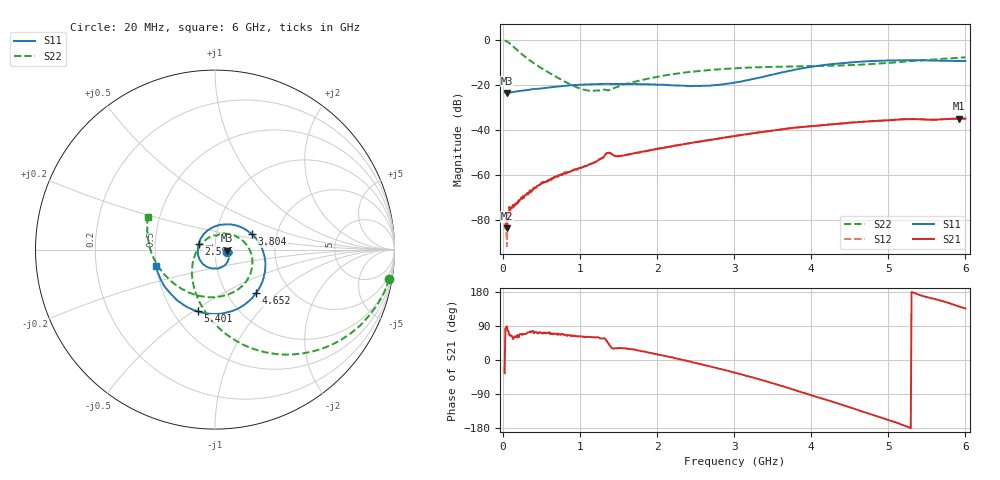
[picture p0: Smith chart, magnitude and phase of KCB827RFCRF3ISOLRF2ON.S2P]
!Agilent Technologies,E5071B,JP1KK00126,A.08.11
!Date: Tue May 06 07:21:44 2014
!Data & Calibration Information:
!Freq	S11:SOLT2(ON)	S21:SOLT2(ON)	S12:SOLT2(ON)	S22:SOLT2(ON)
# Hz S dB R 50
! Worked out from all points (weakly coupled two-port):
!   600 points, 20 MHz to 6 GHz, reference 50 ohm
!   highest |S21| = -34.86 dB at 5.92 GHz (marker M1); lowest = -83.7 dB at 49.95 MHz (marker M2)
!   lowest |S11| = -23.4 dB at 49.95 MHz (marker M3), VSWR 1.14, Z = 57.2 - j0.642 ohm
!   |S11| at or under -10 dB: start of sweep to 4.461 GHz
!   |S22| runs from -22.6 to -0.1 dB; largest |S21 - S12| = 0.00014
!   S11 on the Smith chart (normalised r, x): 20 MHz: 1.14, -0.03; 2.596 GHz: 0.83, +0.05; 3.804 GHz: 1.49, +0.27; 4.652 GHz: 1.36, -0.74; 5.401 GHz: 0.66, -0.52; 6 GHz: 0.50, -0.10
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2e7  -23.20 -12.7  -82.57 -34.7  -84.04 -22.6  -0.13 -9.6
4.994992e7  -23.43 -4.8  -83.69 88.9  -91.59 17.7  -0.60 -23.3
8.988314e7  -23.29 -3.3  -74.31 64.0  -78.09 80.3  -1.54 -39.4
1.397997e8  -23.01 -3.6  -73.86 59.9  -74.07 63.1  -3.04 -56.1
2.196661e8  -22.55 -5.7  -70.89 68.2  -71.16 69.3  -5.50 -75.9
3.294825e8  -22.12 -12.0  -68.46 73.3  -67.84 77.3  -8.55 -95.6
5.690818e8  -21.21 -25.9  -62.47 71.8  -62.66 69.4  -13.93 -129.2
1.018331e9  -19.75 -58.4  -56.70 62.5  -56.49 63.0  -21.78 157.1
1.19803e9  -19.55 -72.7  -54.10 59.7  -54.22 60.3  -22.44 116.5
1.357763e9  -19.45 -85.7  -50.19 45.8  -50.16 45.6  -22.24 84.8
1.517496e9  -19.46 -99.3  -51.44 31.6  -51.50 32.1  -20.35 66.8
2.016661e9  -19.82 -141.6  -48.24 14.4  -48.21 14.7  -16.20 21.7
2.595693e9  -20.27 161.2  -44.83 -12.5  -44.84 -12.5  -13.51 -11.5
3.014992e9  -18.80 110.5  -42.58 -33.9  -42.57 -33.8  -12.50 -33.1
3.444274e9  -15.69 58.7  -40.42 -57.9  -40.39 -58.2  -11.92 -55.0
3.803673e9  -13.00 22.3  -38.86 -80.7  -38.84 -80.6  -11.68 -74.9
4.013322e9  -11.78 3.8  -38.20 -93.8  -38.19 -94.2  -11.59 -87.6
4.652254e9  -9.54 -46.9  -36.32 -135.2  -36.32 -135.3  -10.86 -129.4
5.011653e9  -9.00 -73.8  -35.58 -159.1  -35.57 -159.3  -10.08 -153.1
5.401002e9  -8.93 -105.8  -35.17 171.9  -35.16 171.7  -8.99 -176.5
5.920134e9  -9.28 -155.8  -34.86 141.0  -34.87 141.0  -7.79 157.7
6e9  -9.28 -164.2  -34.88 136.0  -34.86 135.8  -7.64 153.8
